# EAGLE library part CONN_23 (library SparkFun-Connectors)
Multi connection point. Often used as Generic Header-pin footprint for 0.1 inch spaced/style header connections On any of the 0.1 inch spaced packages, you can populate with these: Break Away Headers - Straight (PRT-00116) Break Away Male Headers - Right Angle (PRT-00553) Female Headers (PRT-00115) Break Away Headers - Machine Pin (PRT-00117) Break Away Female Headers - Swiss Machine Pin (PRT-00743) For SCREWTERMINALS and SPRING TERMINALS visit here: Screw Terimnals on SparkFun.com (5mm/3.5mm/2.54mm spacing) This device is also useful as a general connection point to wire up your design to another part of your project. Our various solder wires solder well into these plated through hole pads. Hook-Up Wire - Assortment (Stranded, 22 AWG) (PRT-11375) Hook-Up Wire - Assortment (Solid Core, 22 AWG) (PRT-11367) View the entire wire category on our website here Special notes: Molex polarized connector foot print use with SKU : PRT-08231 with associated crimp pins and housings. 1MM SMD Version SKU: PRT-10208 NOTES ON THE VARIANTS LOCK and LOCK_LONGPADS... This footprint was designed to help hold the alignment of a through-hole component (i.e. 6-pin header) while soldering it into place. You may notice that each hole has been shifted either up or down by 0.005 of an inch from it's more standard position (which is a perfectly straight line). This slight alteration caused the pins (the squares in the middle) to touch the edges of the holes. Because they are alternating, it causes a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
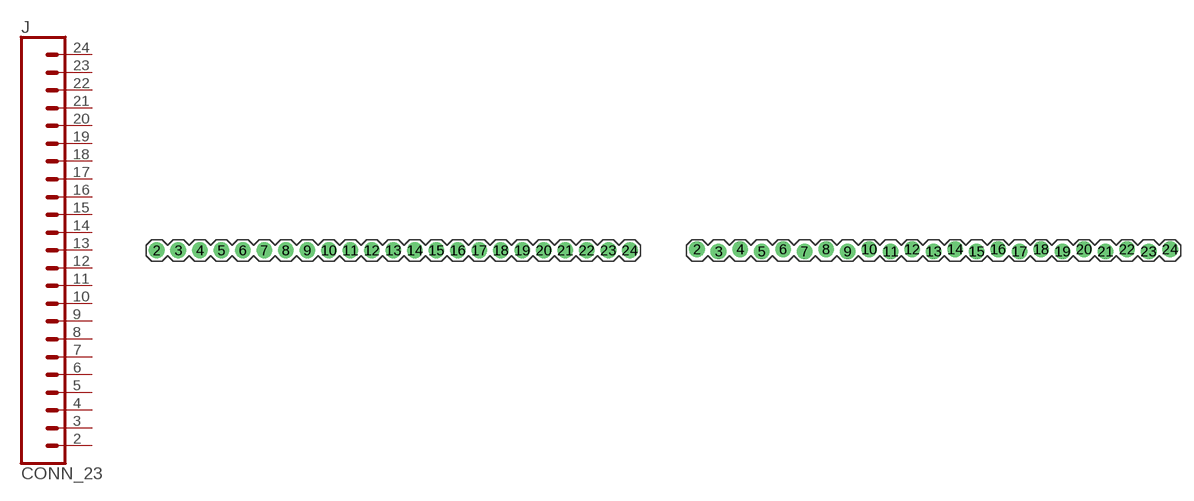
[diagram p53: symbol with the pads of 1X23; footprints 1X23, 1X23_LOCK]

Designator prefix J

## CONN_23  [1X23]
2  2  pas
3  3  pas
4  4  pas
5  5  pas
6  6  pas
7  7  pas
8  8  pas
9  9  pas
10  10  pas
11  11  pas
12  12  pas
13  13  pas
14  14  pas
15  15  pas
16  16  pas
17  17  pas
18  18  pas
19  19  pas
20  20  pas
21  21  pas
22  22  pas
23  23  pas
24  24  pas

## CONN_23LOCK  [1X23_LOCK]
Pads as for 1X23

## CONN_23LONGPADS  [1X23_LONGPADS]
Pads as for 1X23

## Footprint 1X23 (pad centres in mm)
Plated Through Hole -23 Pin Specifications: Pin count:23 Pin pitch:0.1" Example device(s): CONN_23
drill 1.016 pad 1.88: 2 -26.67,0; 3 -24.13,0; 4 -21.59,0; 5 -19.05,0; 6 -16.51,0; 7 -13.97,0; 8 -11.43,0; 9 -8.89,0; 10 -6.35,0; 11 -3.81,0; 12 -1.27,0; 13 1.27,0; 14 3.81,0; 15 6.35,0; 16 8.89,0; 17 11.43,0; 18 13.97,0; 19 16.51,0; 20 19.05,0; 21 21.59,0; 22 24.13,0; 23 26.67,0; 24 29.21,0

## Footprint 1X23_LOCK (pad centres in mm)
Plated Through Hole -23 Pin Locking Footprint Holes are offset 0.005" from center, to hold pins in place while soldering Specifications: Pin count:23 Pin pitch:0.1" Example device(s): CONN_23
drill 1.016 pad 1.88: 2 -26.67,0.127; 3 -24.13,-0.127; 4 -21.59,0.127; 5 -19.05,-0.127; 6 -16.51,0.127; 7 -13.97,-0.127; 8 -11.43,0.127; 9 -8.89,-0.127; 10 -6.35,0.127; 11 -3.81,-0.127; 12 -1.27,0.127; 13 1.27,-0.127; 14 3.81,0.127; 15 6.35,-0.127; 16 8.89,0.127; 17 11.43,-0.127; 18 13.97,0.127; 19 16.51,-0.127; 20 19.05,0.127; 21 21.59,-0.127; 22 24.13,0.127; 23 26.67,-0.127; 24 29.21,0.127

## Footprint 1X23_LONGPADS (pad centres in mm)
Plated Through Hole -23 Pin Long Pads Specifications: Pin count:23 Pin pitch:0.1" Example device(s): CONN_23
drill 1.118 pad 1.88 long: 2 -26.67,0; 3 -24.13,0; 4 -21.59,0; 5 -19.05,0; 6 -16.51,0; 7 -13.97,0; 8 -11.43,0; 9 -8.89,0; 10 -6.35,0; 11 -3.81,0; 12 -1.27,0; 13 1.27,0; 14 3.81,0; 15 6.35,0; 16 8.89,0; 17 11.43,0; 18 13.97,0; 19 16.51,0; 20 19.05,0; 21 21.59,0; 22 24.13,0; 23 26.67,0; 24 29.21,0; 25 31.75,0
